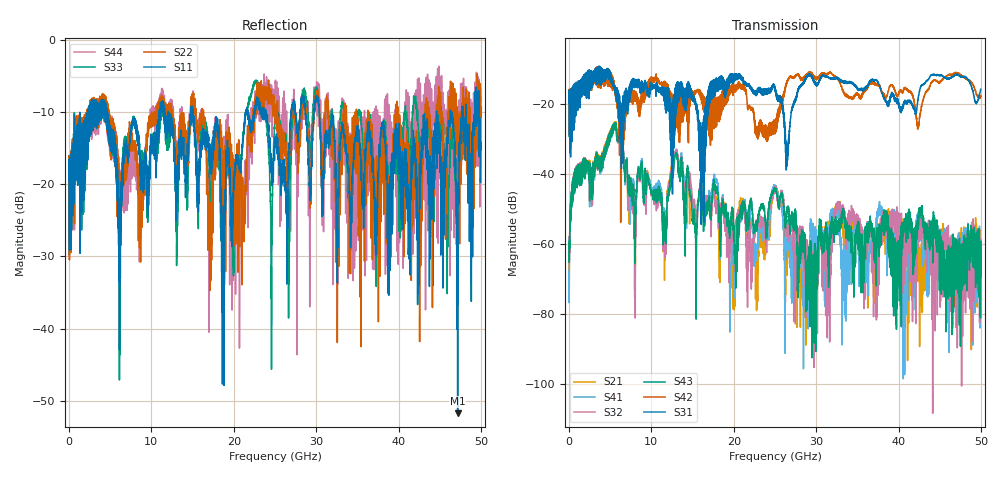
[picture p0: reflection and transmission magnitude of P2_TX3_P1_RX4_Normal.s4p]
!Keysight Technologies,N5225B,MY57041031,A.13.20.10
!Date: Friday, May 31, 2019 11:19:55
!Correction: S11(Full 4 Port(1,2,3,4))
!S12(Full 4 Port(1,2,3,4))
!S13(Full 4 Port(1,2,3,4))
!S14(Full 4 Port(1,2,3,4))
!S21(Full 4 Port(1,2,3,4))
!S22(Full 4 Port(1,2,3,4))
!S23(Full 4 Port(1,2,3,4))
!S24(Full 4 Port(1,2,3,4))
!S31(Full 4 Port(1,2,3,4))
!S32(Full 4 Port(1,2,3,4))
!S33(Full 4 Port(1,2,3,4))
!S34(Full 4 Port(1,2,3,4))
!S41(Full 4 Port(1,2,3,4))
!S42(Full 4 Port(1,2,3,4))
!S43(Full 4 Port(1,2,3,4))
!S44(Full 4 Port(1,2,3,4))
!S4P File: Measurements: <S11,S12,S13,S14>,
!<S21,S22,S23,S24>,
!<S31,S32,S33,S34>,
!<S41,S42,S43,S44>:
# Hz S  dB  R 50.0
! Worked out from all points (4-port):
!   5000 points, 10 MHz to 50 GHz, reference 50 ohm
!   strongest paths, dB at 10 MHz, 12.51 GHz, 25.01 GHz, 37.51 GHz, 50 GHz:
!     S31: -19.5, -43.6, -16.0, -13.6, -15.6
!     S42: -19.4, -19.4, -25.6, -14.5, -17.4
!     S43: -61.2, -40.3, -44.0, -57.6, -69.0
!     S32: -61.7, -39.2, -44.2, -74.6, -65.7
!     S41: -67.8, -39.4, -43.7, -51.1, -61.8
!     S21: -57.9, -38.4, -44.3, -58.1, -69.7
!   lowest |S11| = -51.7 dB at 47.18 GHz (marker M1), VSWR 1.01, Z = 49.8 - j0.0792 ohm
!   |S11| at or under -10 dB: 4.63 GHz to 10.95 GHz (6.318 GHz wide, 81.1 % of centre); 15.04 GHz to 21.46 GHz (6.427 GHz wide, 35.2 % of centre); 30.38 GHz to 44.61 GHz (14.23 GHz wide, 37.9 % of centre)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
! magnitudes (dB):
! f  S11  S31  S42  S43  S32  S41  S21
! 10 MHz  -19.6  -19.5  -19.4  -61.2  -61.7  -67.8  -57.9
! 5.51 GHz  -12.8  -15.4  -15.0  -25.4  -25.4  -25.6  -25.1
! 19.93 GHz  -21.2  -14.0  -16.9  -53.4  -57.0  -65.9  -62.5
! 25.12 GHz  -13.6  -16.6  -27.7  -44.1  -43.8  -43.7  -43.8
! 28.45 GHz  -8.2  -13.9  -12.7  -62.5  -61.4  -61.5  -65.0
! 47.18 GHz  -51.7  -11.4  -11.1  -65.3  -65.2  -65.0  -69.2
! 50 GHz  -15.1  -15.6  -17.4  -69.0  -65.7  -61.8  -69.7
